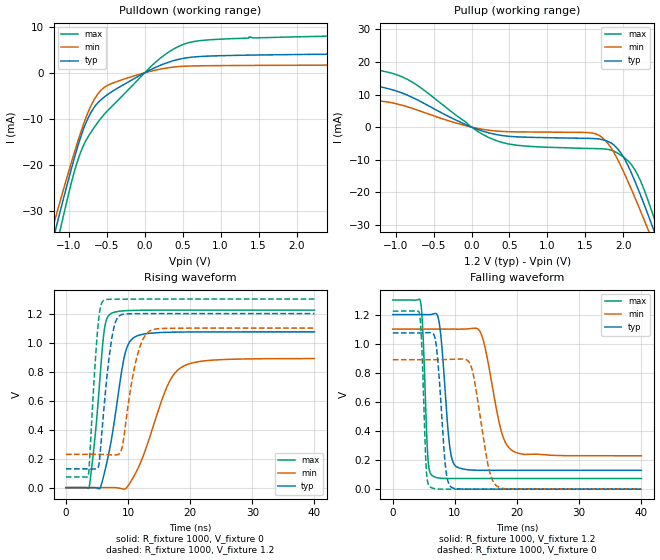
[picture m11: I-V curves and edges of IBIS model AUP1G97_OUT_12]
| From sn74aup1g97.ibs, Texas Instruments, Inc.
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[Model]   AUP1G97_OUT_12
Model_type  Output
Vref =   0
Rref =   1E6
Cref =   30p
Vmeas =   0.6
| variable   typ   min   max
C_comp   2.77pF   2.03pF   3.84pF
| C_pullup   2.95pF   2.03pF   3.84pF
| C_pulldown   2.59pF   2.14pF   3.08pF
[Temperature Range]   40   100   -40
| Ambient temperature   25   85   -40
[Voltage range]   1.2   1.1   1.3
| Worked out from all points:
|   slope of the pulldown table from 0 to 0.18 V, typ, clamps not added: 125 ohm
|   slope of the pullup table from 0 to 0.18 V, typ, clamps not added: 123 ohm
|   rising waveform, R_fixture 1000, V_fixture 0: 20-80 % time 2.4ns typ, 4.38ns min, 1.47ns max; typ from 0 V to 1.07 V
|   falling waveform, R_fixture 1000, V_fixture 1.2: 20-80 % time 1.14ns typ, 2.34ns min, 645ps max; typ from 1.2 V to 0.129 V
|   rising waveform, R_fixture 1000, V_fixture 1.2: 20-80 % time 1.51ns typ, 2.09ns min, 1.07ns max; typ from 0.129 V to 1.2 V
|   falling waveform, R_fixture 1000, V_fixture 0: 20-80 % time 1.05ns typ, 1.99ns min, 600ps max; typ from 1.07 V to 0 V
[Pulldown]
| AUP1G97_OUT_12
|   Voltage   I(typ)   I(min)   I(max)
-3.6V     -203.6mA   -186.6mA   -224.6mA
-1.215V   -36.77mA   -33.88mA   -41.55mA
-1.165V   -33.49mA   -30.92mA   -37.89mA
-1.12V    -30.57mA   -28.28mA   -34.63mA
-1.08V    -28mA      -25.95mA   -31.76mA
-930mV    -18.76mA   -17.53mA   -21.68mA
-820mV    -12.87mA   -11.86mA   -16.33mA
-695mV    -8.261mA   -6.747mA   -12.62mA
-580mV    -5.938mA   -3.862mA   -9.962mA
160mV     1.298mA    643.5uA    2.533mA
610mV     3.376mA    1.481mA    6.659mA
7.2V      4.761mA    1.852mA    9.574mA
[Pullup]
| AUP1G97_OUT_12
|   Voltage   I(typ)   I(min)   I(max)
-3.6V     26.64mA    8.226mA    37.8mA
-3.065V   21.41mA    10.49mA    30.92mA
-2.05V    13.06mA    7.529mA    19.66mA
-955mV    10.79mA    6.951mA    15.81mA
400mV     -2.561mA   -1.314mA   -4.679mA
1.61V     -3.491mA   -1.891mA   -6.566mA
1.87V     -5.387mA   -7.563mA   -7.321mA
2.095V    -13.49mA   -18.49mA   -11.17mA
2.33V     -27.16mA   -31.66mA   -22.8mA
2.44V     -34.07mA   -38.08mA   -30.25mA
2.51V     -38.55mA   -42.22mA   -35.17mA
7.2V      -371mA     -348.5mA   -398.6mA
[Ramp]
| AUP1G97_OUT_12
| variable   typ   min   max
dV/dt_r   0.65/2.42E-09   0.54/4.43E-09   0.74/1.48E-09
dV/dt_f   0.65/1.15E-09   0.53/2.35E-09   0.74/6.52E-10
R_load = 1000
[Rising Waveform]
| AUP1G97_OUT_12
R_fixture =   1000
C_fixture =   0
L_fixture =   0
V_fixture =   0
V_fixture_min = 0
V_fixture_max = 0
|   Time   V(typ)   V(min)   V(max)
0s        17.04nV    106.6nV    899pV
3.735ns   298.9uV    -5.61uV    5.073mV
4.765ns   -381.4uV   24.11uV    387.3mV
6.09ns    83.95mV    338.1uV    1.059V
7.14ns    289.6mV    178.9uV    1.197V
9.405ns   903.5mV    -10.59mV   1.219V
11.09ns   1.039V     89.97mV    1.222V
16.25ns   1.071V     693.4mV    1.224V
18.54ns   1.073V     827.9mV    1.224V
40ns      1.074V     889.7mV    1.224V
[Falling Waveform]
| AUP1G97_OUT_12
R_fixture =   1000
C_fixture =   0
L_fixture =   0
V_fixture =   1.2
V_fixture_min = 1.1
V_fixture_max = 1.3
|   Time   V(typ)   V(min)   V(max)
0s        1.2V       1.1V       1.3V
4.45ns    1.2V       1.1V       1.29V
5.625ns   1.2V       1.1V       230.2mV
6.335ns   1.202V     1.1V       93.62mV
7.485ns   1.139V     1.1V       75.83mV
9.1ns     313.1mV    1.1V       73.66mV
10.19ns   155.3mV    1.1V       73.56mV
14.16ns   129.8mV    1.073V     73.54mV
19.22ns   129.5mV    265.1mV    73.54mV
40ns      129.5mV    229.3mV    73.54mV
[Rising Waveform]
| AUP1G97_OUT_12
R_fixture =   1000
C_fixture =   0
L_fixture =   0
V_fixture =   1.2
V_fixture_min = 1.1
V_fixture_max = 1.3
|   Time   V(typ)   V(min)   V(max)
0s        129.5mV    229.3mV    73.54mV
3.595ns   129.5mV    229.4mV    83.32mV
5.1ns     134.2mV    229.4mV    1.088V
6.045ns   514.3mV    228.4mV    1.289V
7.13ns    956.9mV    226.3mV    1.299V
8.11ns    1.156V     225.5mV    1.3V
9.075ns   1.194V     283.6mV    1.3V
11.48ns   1.199V     910.5mV    1.3V
13.49ns   1.2V       1.08V      1.3V
40ns      1.2V       1.1V       1.3V
[Falling Waveform]
| AUP1G97_OUT_12
R_fixture =   1000
C_fixture =   0
L_fixture =   0
V_fixture =   0
V_fixture_min = 0
V_fixture_max = 0
|   Time   V(typ)   V(min)   V(max)
0s        1.074V     889.8mV    1.224V
4.28ns    1.074V     889.8mV    1.209V
5.375ns   1.075V     889.8mV    147.5mV
5.99ns    1.076V     889.7mV    15.21mV
6.95ns    1V         889.7mV    1.966mV
8.465ns   159.6mV    891mV      52.19uV
9.42ns    13.41mV    892.5mV    7.422uV
12.6ns    67.75uV    844.3mV    71nV
16.81ns   747.1nV    19.55mV    -47.31nV
40ns      -8.519nV   103.3nV    -42.24nV
